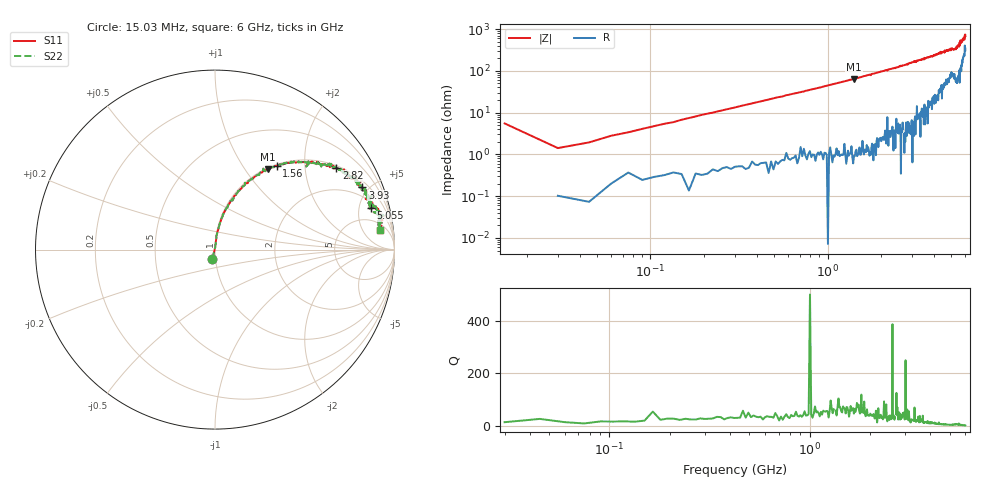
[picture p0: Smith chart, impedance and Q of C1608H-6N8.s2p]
!	Network	Analyzer	HP8753E.07.74:	Oct	30	2002	Serial	No.	JP38451487
!	Hewlett-Packard
!	7	Sep	2009	10:13:58
!	Frequency	S11	S21	S12	S22
#	HZ	S	RI	R	50
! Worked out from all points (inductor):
!   400 points, 15.03 MHz to 6 GHz, reference 50 ohm
!   read as one part in series: L = 7.12 nH near 45.03 MHz
!   highest Q = 70.4 at 1.41 GHz (marker M1), where L = 7.25 nH
!   S11 on the Smith chart (normalised r, x): 15.03 MHz: 0.96, -0.10; 1.56 GHz: 1.03, +1.44; 2.82 GHz: 1.07, +2.91; 3.93 GHz: 1.36, +4.56; 5.055 GHz: 2.72, +6.59; 6 GHz: 8, +12
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1.502992e7  -0.0153 -0.0533  1.02 0.0533  1.02 0.0533  -0.0153 -0.0533
3.002985e7  0.00144 0.0141  0.999 -0.0141  0.999 -0.0141  0.00144 0.0141
6.00297e7  0.00253 0.0277  0.997 -0.0277  0.997 -0.0277  0.00253 0.0277
1.200294e8  0.00613 0.0535  0.994 -0.0535  0.994 -0.0535  0.00613 0.0535
2.850286e8  0.0203 0.124  0.98 -0.124  0.98 -0.124  0.0203 0.124
5.850271e8  0.0727 0.24  0.927 -0.24  0.927 -0.24  0.0727 0.24
1.020025e9  0.176 0.369  0.824 -0.369  0.824 -0.369  0.176 0.369
1.410023e9  0.295 0.449  0.705 -0.449  0.705 -0.449  0.295 0.449
1.560022e9  0.343 0.466  0.657 -0.466  0.657 -0.466  0.343 0.466
2.01002e9  0.481 0.489  0.519 -0.489  0.519 -0.489  0.481 0.489
2.820016e9  0.676 0.456  0.324 -0.456  0.324 -0.456  0.676 0.456
3.015015e9  0.72 0.447  0.28 -0.447  0.28 -0.447  0.72 0.447
3.93001e9  0.821 0.346  0.179 -0.346  0.179 -0.346  0.821 0.346
4.00501e9  0.837 0.337  0.163 -0.337  0.163 -0.337  0.837 0.337
5.010005e9  0.863 0.236  0.137 -0.236  0.137 -0.236  0.863 0.236
5.055005e9  0.87 0.23  0.13 -0.23  0.13 -0.23  0.87 0.23
5.535002e9  0.884 0.209  0.116 -0.209  0.116 -0.209  0.884 0.209
5.565002e9  0.939 0.19  0.0605 -0.19  0.0605 -0.19  0.939 0.19
5.595002e9  0.901 0.199  0.0989 -0.199  0.0989 -0.199  0.901 0.199
5.625002e9  0.933 0.163  0.0674 -0.163  0.0674 -0.163  0.933 0.163
5.715001e9  0.915 0.173  0.0854 -0.173  0.0854 -0.173  0.915 0.173
6e9  0.918 0.109  0.0821 -0.109  0.0821 -0.109  0.918 0.109
